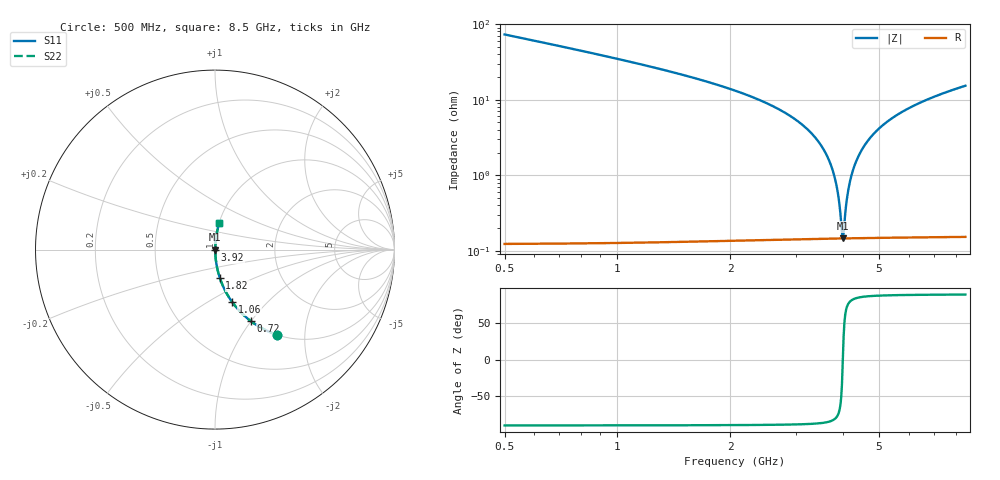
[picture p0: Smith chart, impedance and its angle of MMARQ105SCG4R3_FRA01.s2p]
! MMARQ105SCG4R3_FRA01  S-PARAMETER MODEL  ( General Type )
! Model Generated by TAIYO YUDEN Corporation (http://www.ty-top.com)
! Version 1.0
! TAIYO YUDEN Control No. 200326
! Copyright(c) 2020 TAIYO YUDEN CO.,LTD. All Rights Reserved.
! Product Description (link to TY-COMPAS)
! https://ds.yuden.co.jp/TYCOMPAS/or/detail?pn=MMARQ105SCG4R3BFRA01&u=M
! Products Name : Multilayer Ceramic Capacitors
! Characteristics :
!  Capacitance : 4.3 pF , Rated Voltage : 250V , TCC : CG / C0G
!  Case Size : 1.0 x 0.5 / 0.039 x 0.02 [mm/inch] , Thickness : 0.5 / 0.02 [mm/inch]
!  (Conditions: Temperature = 25 degC , DC Bias Current/Voltage = 0A / 0V)
! External Node Assignments :
!  1  o---| |---o  2
! GND o---------o GND
! Frequency Range : 500MHz  -  8.5GHz  [ 401 STEP ]
# MHz S RI R 50
! Freq[MHz].  S11 Real  S11 Imag  S21 Real  S21 Imag  S12 Real  S12 Imag  S22 Real  S22 Imag
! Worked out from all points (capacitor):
!   401 points, 500 MHz to 8.5 GHz, reference 50 ohm
!   read as one part in series: C = 4.3 pF near 540 MHz
!   lowest |Z| = 146 mohm at 4 GHz (marker M1)
!   series resonance near 4 GHz, so ESL is about 370 pH
!   S11 on the Smith chart (normalised r, x): 500 MHz: 1.00, -1.46; 720 MHz: 1.00, -1.00; 1.06 GHz: 1.00, -0.65; 1.82 GHz: 1.00, -0.32; 3.92 GHz: 1.00, -0.01; 8.5 GHz: 1.00, +0.31
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500  0.3476 -0.4753  0.6524 0.4753  0.6524 0.4753  0.3476 -0.4753
720  0.1993 -0.3982  0.8007 0.3982  0.8007 0.3982  0.1993 -0.3982
1060  0.0964 -0.2932  0.9036 0.2932  0.9036 0.2932  0.0964 -0.2932
1820  0.0266 -0.1569  0.9734 0.1569  0.9734 0.1569  0.0266 -0.1569
1840  0.0258 -0.1544  0.9742 0.1544  0.9742 0.1544  0.0258 -0.1544
2660  0.00737 -0.077  0.9926 0.077  0.9926 0.077  0.00737 -0.077
3180  0.00325 -0.0426  0.9967 0.0426  0.9967 0.0426  0.00325 -0.0426
3460  0.00216 -0.0269  0.9978 0.0269  0.9978 0.0269  0.00216 -0.0269
3680  0.00169 -0.0154  0.9983 0.0154  0.9983 0.0154  0.00169 -0.0154
3820  0.00152 -0.00852  0.9985 0.00852  0.9985 0.00852  0.00152 -0.00852
3920  0.00147 -0.00374  0.9985 0.00374  0.9985 0.00374  0.00147 -0.00374
3960  0.00146 -0.00187  0.9985 0.00187  0.9985 0.00187  0.00146 -0.00187
4000  0.00146 -1.66e-05  0.9985 1.66e-05  0.9985 1.66e-05  0.00146 -1.66e-05
4040  0.00146 0.00182  0.9985 -0.00182  0.9985 -0.00182  0.00146 0.00182
4120  0.00149 0.00544  0.9985 -0.00544  0.9985 -0.00544  0.00149 0.00544
4200  0.00154 0.00899  0.9985 -0.00899  0.9985 -0.00899  0.00154 0.00899
4320  0.00167 0.0142  0.9983 -0.0142  0.9983 -0.0142  0.00167 0.0142
4500  0.00195 0.0218  0.9981 -0.0218  0.9981 -0.0218  0.00195 0.0218
5020  0.00327 0.0422  0.9967 -0.0422  0.9967 -0.0422  0.00327 0.0422
5840  0.00659 0.0711  0.9934 -0.0711  0.9934 -0.0711  0.00659 0.0711
7180  0.0144 0.1127  0.9856 -0.1127  0.9856 -0.1127  0.0144 0.1127
8500  0.0243 0.1491  0.9757 -0.1491  0.9757 -0.1491  0.0243 0.1491
